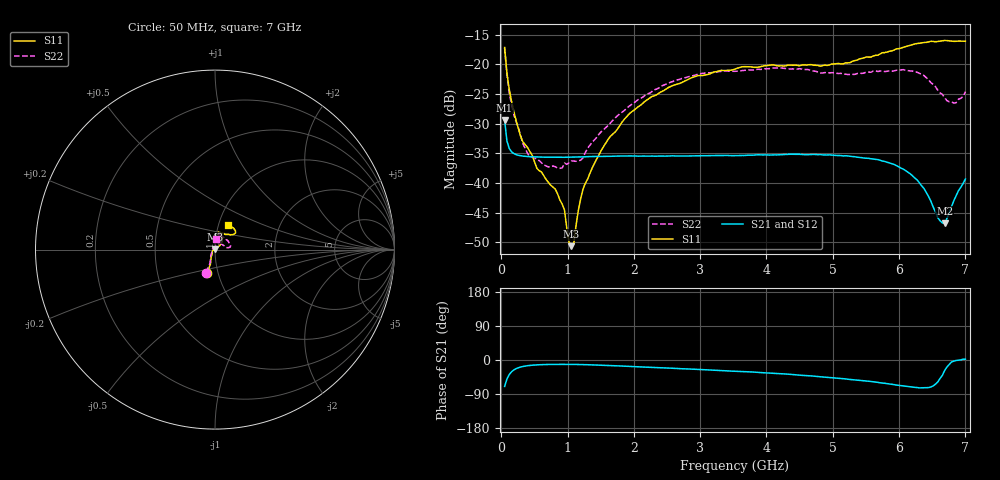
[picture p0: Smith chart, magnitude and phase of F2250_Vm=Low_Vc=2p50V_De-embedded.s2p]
! Integrated Device Technology
! Corporate Headquarters
! 6024 Silver Creek Valley Road
! San Jose, CA 95138  USA
! Phone:  1-408-284-8200
! Toll Free:  1-800-223-1366
! Webpage:  http://www.idt.com/
! Timing and RF Division
! 515 Groton Road, Suite 102
! Westford, MA 01886-6024
! Device:  F2250
! Description: Voltage Variable RF Attenuator
! Frequency:  50.0 -  6000.00 MHz
! Package:  3x3 mm Thin QFN Plastic Package: 16 pin
! Ports:  2 RF, 3 DC
!  Pin  1  = GND
!  Pin  2  = NC
!  Pin  3  = RF1  = Port 1
!  Pin  4  = NC
!  Pin  5  = GND
!  Pin  6  = GND
!  Pin  7  = GND
!  Pin  8  = GND
!  Pin  9  = NC
!  Pin 10  = RF2  = Port 2
!  Pin 11  = NC
!  Pin 12  = GND
!  Pin 13  = GND
!  Pin 14  = VCNTRL
!  Pin 15  = VDD
!  Pin 16  = VMODE
! Vcntrl:  2.500 Volts
! Vmode:  +0.000 Volts
! Vdd:  +3.30  Volts
! Current:  1.176 mA
! Data:  The device was measured on a the F2250 evaluation board which has
!  individual transmission lines to the RF pins.  Data was collected
!  using a calibrated network analyzer.  The evaluation board was
!  de-embedded using a TRL calibration technique.
!  The reference plane is the edge of the package pin.
! Misc:  SN 10
!  Action Tracker AT0258
! Date Measured:  2014-11-26
! Date:  2015-10-15  MJV
! Note:
!  Integrated Device Technology supplies this data as a sample of measured
!  data at the package pin for this product.  Your particular data for this
!  product may vary.
!  Data was taken at 25 degrees C.
!  Integrated Device Technology reserves the right to change this data at anytime.
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# GHz S dB R 50
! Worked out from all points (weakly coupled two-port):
!   201 points, 50 MHz to 7 GHz, reference 50 ohm
!   highest |S21| = -29.41 dB at 50 MHz (marker M1); lowest = -46.8 dB at 6.687 GHz (marker M2)
!   lowest |S11| = -50.7 dB at 1.058 GHz (marker M3), VSWR 1.01, Z = 49.8 + j0.244 ohm
!   |S11| at or under -10 dB: start of sweep to end of sweep
!   |S22| runs from -37.5 to -17.3 dB; largest |S21 - S12| = 5.9e-05
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0.05  -17.18 -108.6  -29.41 -69.8  -29.41 -69.8  -17.28 -111.0
0.08475  -21.44 -107.4  -32.92 -50.4  -32.92 -50.3  -21.75 -110.2
0.15425  -26.23 -116.6  -34.76 -31.2  -34.75 -31.1  -26.82 -122.4
0.29325  -32.21 -127.8  -35.43 -18.5  -35.43 -18.5  -32.11 -137.5
0.3975  -34.08 -141.6  -35.56 -15.0  -35.56 -15.0  -35.06 -160.5
0.91875  -43.58 158.2  -35.69 -11.5  -35.69 -11.5  -37.48 133.4
0.9535  -44.60 169.7  -35.69 -11.5  -35.68 -11.5  -36.66 131.2
1.023  -50.02 143.9  -35.68 -11.6  -35.67 -11.6  -36.60 116.0
1.05775  -50.67 123.2  -35.67 -11.6  -35.67 -11.6  -36.29 110.9
1.0925  -50.35 90.1  -35.66 -11.7  -35.66 -11.7  -36.32 106.3
1.162  -44.65 56.7  -35.64 -11.9  -35.64 -11.9  -36.24 95.6
1.2315  -41.13 44.1  -35.61 -12.1  -35.61 -12.1  -35.79 85.9
1.6485  -32.12 41.9  -35.52 -14.6  -35.52 -14.6  -29.88 64.6
1.9265  -28.40 41.3  -35.47 -16.9  -35.47 -16.9  -27.09 56.7
2.37825  -24.87 47.3  -35.48 -20.3  -35.48 -20.3  -23.99 56.8
3.525  -20.80 72.5  -35.40 -29.5  -35.40 -29.5  -21.19 74.8
4.7065  -20.17 72.3  -35.20 -42.6  -35.21 -42.5  -21.14 72.3
5.85325  -17.81 40.5  -36.64 -63.2  -36.64 -63.3  -21.13 23.0
6.27025  -16.50 40.1  -39.50 -72.6  -39.50 -72.6  -21.35 9.6
6.68725  -15.99 48.8  -46.85 -27.6  -46.81 -27.4  -25.64 28.5
6.861  -16.13 55.1  -42.17 -1.2  -42.14 -1.2  -26.47 58.0
7  -16.13 63.2  -39.34 1.9  -39.31 1.8  -24.62 83.1
